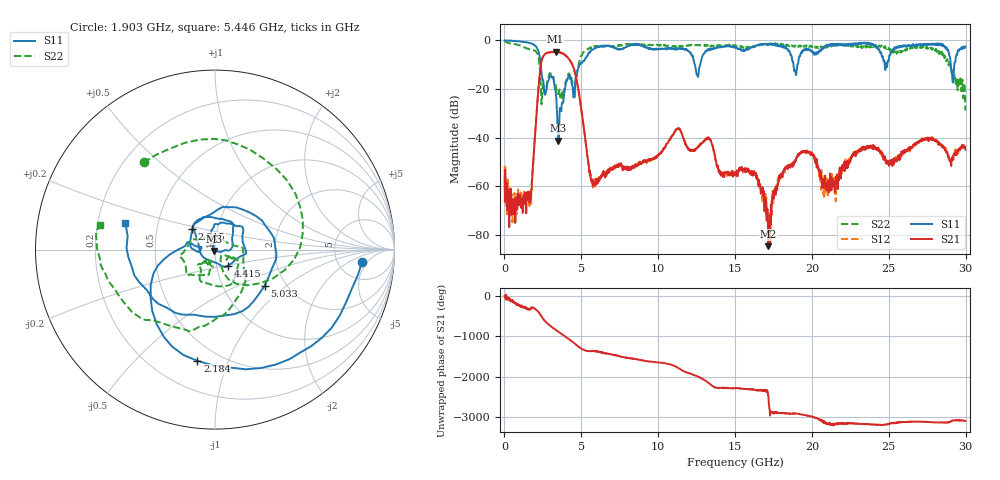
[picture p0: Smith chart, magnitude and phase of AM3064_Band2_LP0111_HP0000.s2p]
# Hz S DB R 50.0
!freq dBS11 angS11 dBS21 angS21 dBS12 angS12 dBS22 angS22
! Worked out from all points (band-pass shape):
!   1600 points, 10 MHz to 29.98 GHz, reference 50 ohm
!   highest |S21| = -4.60 dB at 3.328 GHz (marker M1); lowest = -84.6 dB at 17.16 GHz (marker M2)
!   |S21| within 3 dB of the highest: 2.45 GHz to 4.187 GHz (1.737 GHz wide, 52.3 % of centre)
!   lowest |S11| = -41.2 dB at 3.515 GHz (marker M3), VSWR 1.02, Z = 49.5 - j0.716 ohm
!   |S11| at or under -10 dB: 2.36 GHz to 4.889 GHz (2.529 GHz wide, 69.8 % of centre); 12.38 GHz to 12.72 GHz (343.2 MHz wide, 2.73 % of centre); 18.8 GHz to 19.05 GHz (252.6 MHz wide, 1.34 % of centre)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
!   |S22| runs from -28.8 to -0.2 dB; largest |S21 - S12| = 0.019
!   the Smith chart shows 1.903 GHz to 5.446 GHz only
!   S11 on the Smith chart (normalised r, x): 1.903 GHz: 8.57, -3.74; 2.184 GHz: 0.38, -0.78; 2.915 GHz: 0.76, +0.18; 4.415 GHz: 1.13, -0.21; 5.033 GHz: 1.56, -0.72; 5.446 GHz: 0.32, +0.13
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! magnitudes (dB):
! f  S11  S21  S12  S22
! 10 MHz  0.0  -55.6  -51.8  -0.2
! 1.584 GHz  -1.0  -63.7  -67.1  -3.5
! 1.903 GHz  -1.7  -46.2  -46.6  -4.1
! 2.184 GHz  -4.1  -21.9  -21.8  -6.1
! 2.915 GHz  -15.3  -4.9  -4.9  -14.0
! 3.328 GHz  -20.9  -4.6  -4.7  -18.5
! 3.515 GHz  -41.2  -4.8  -4.7  -21.8
! 4.415 GHz  -18.8  -10.0  -10.0  -16.7
! 5.015 GHz  -9.5  -29.0  -28.8  -6.3
! 5.033 GHz  -9.3  -29.6  -29.7  -6.1
! 5.446 GHz  -5.7  -50.0  -49.8  -3.7
! 10 GHz  -3.6  -46.9  -47.2  -1.9
! 11.31 GHz  -3.2  -36.4  -36.2  -2.7
! 15 GHz  -2.7  -55.4  -55.0  -2.0
! 16.34 GHz  -2.3  -54.9  -54.6  -2.4
! 17.16 GHz  -1.6  -84.6  -77.9  -1.5
! 18.25 GHz  -3.2  -52.5  -52.9  -1.9
! 19.99 GHz  -4.4  -46.9  -46.4  -2.2
! 20.87 GHz  -2.3  -59.9  -58.1  -3.0
! 25 GHz  -8.0  -50.4  -50.5  -3.1
! 28.31 GHz  -1.7  -42.5  -42.9  -4.6
! 29.98 GHz  -2.4  -44.9  -44.0  -28.8
